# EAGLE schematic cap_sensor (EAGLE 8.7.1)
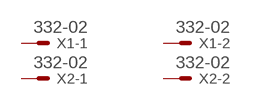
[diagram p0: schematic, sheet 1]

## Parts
X1  332-02  [332-02]
X2  332-02  [332-02]
Unconnected: X1.1 X1.2 X2.1 X2.2

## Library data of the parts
X1 X2 = con-garry:332-02: 2 Pin - 2mm Dual Row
